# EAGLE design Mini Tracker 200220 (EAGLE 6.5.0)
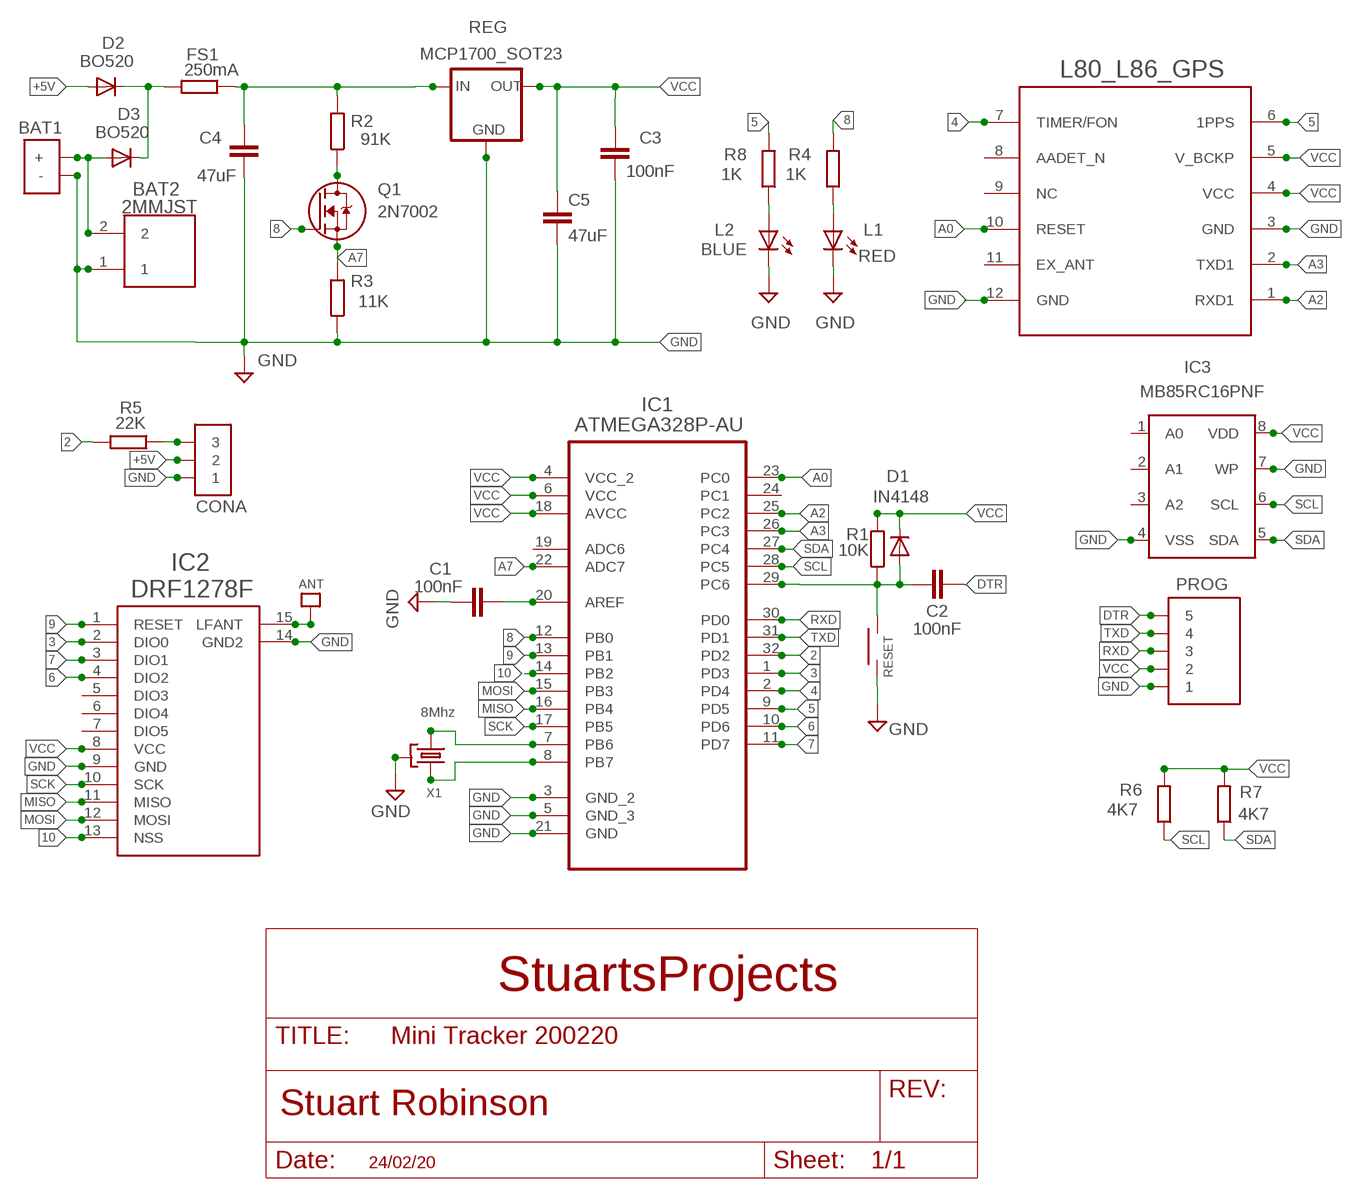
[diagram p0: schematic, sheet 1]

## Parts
ANT  SINGLEPAD  [SINGLEPAD]
BAT1  BATPADS2  [BATPADS]
BAT2  2MMJST  [2MMJST]
C1  100nF  C805_REDUCED  [C0805_REDUCED]
C2  100nF  C805_REDUCED  [C0805_REDUCED]
C3  100nF  C805_REDUCED  [C0805_REDUCED]
C4  47uF  C-EUC1206  [C1206]
C5  47uF  C-EUC1206  [C1206]
CONA  3X1  [3X1]
D1  IN4148  DIODE-SOD123  [SOD123]
D2  BO520  DIODE-SOD123  [SOD123]
D3  BO520  DIODE-SOD123  [SOD123]
FS1  250mA  R-EU_R1206  [R1206]
IC1  ATMEGA328P-AU  [QFP80P900X900X120-32N]
IC2  DRF1278F  DRF1278F_SMT  [DRF1278_SMT]
IC3  MB85RC16PNF  24L256  [SOIC08@1]
L1  RED  LEDCHIPLED_0805  [CHIPLED_0805]
L2  BLUE  LEDCHIPLED_0805  [CHIPLED_0805]
L80_L86_GPS  L80_L86  L80_GNSS_MODULE  [L80_PACKAGE]
PROG  5X1  [5X1]
Q1  2N7002  [SOT23]
R1  10K  R0805_REDUCED  [R0805_REDUCED]
R2  91K  R0805_REDUCED  [R0805_REDUCED]
R3  11K  R0805_REDUCED  [R0805_REDUCED]
R4  1K  R0805_REDUCED  [R0805_REDUCED]
R5  22K  R0805_REDUCED  [R0805_REDUCED]
R6  4K7  R0805_REDUCED  [R0805_REDUCED]
R7  4K7  R0805_REDUCED  [R0805_REDUCED]
R8  1K  R0805_REDUCED  [R0805_REDUCED]
REG  MCP1700_SOT23  [SOT23]
RESET  SMTSWITCH_4_X_3  [SMTSWITCH_4_X_3]
X1  8Mhz  SMTRESONATOR3  [SMTRESONATOR3]

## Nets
2: IC1.32(PD2) R5.2
3: IC1.1(PD3) IC2.2(DIO0)
4: IC1.2(PD4) L80_L86_GPS.7(TIMER/FON)
5: IC1.9(PD5) L80_L86_GPS.6(1PPS) R8.2
6: IC1.10(PD6) IC2.4(DIO2)
7: IC1.11(PD7) IC2.3(DIO1)
8: IC1.12(PB0) Q1.1(G) R4.2
9: IC1.13(PB1) IC2.1(RESET)
10: IC1.14(PB2) IC2.13(NSS)
+5V [POWER]: CONA.2 D2.A
A0: IC1.23(PC0) L80_L86_GPS.10(RESET)
A2: IC1.25(PC2) L80_L86_GPS.1(RXD1)
A3: IC1.26(PC3) L80_L86_GPS.2(TXD1)
A7: IC1.22(ADC7) Q1.2(S) R3.2
DTR: C2.2 PROG.5
GND [POWER]: BAT1.BAT-V(-) BAT2.1 C1.2 C3.2 C4.2 C5.2 CONA.1 IC1.3(GND_2) IC1.5(GND_3) IC1.21(GND) IC2.9(GND) IC2.14(GND2) IC3.4(VSS) IC3.7(WP) L1.C L2.C L80_L86_GPS.3(GND) L80_L86_GPS.12(GND) PROG.1 R3.1 REG.1(GND) RESET.1 X1.G(GND)
MISO: IC1.16(PB4) IC2.11(MISO)
MOSI: IC1.15(PB3) IC2.12(MOSI)
N$1: IC1.8(PB7) X1.X2
N$2: IC1.7(PB6) X1.X1
N$3: C1.1 IC1.20(AREF)
N$4: ANT.P$1 IC2.15(LFANT)
N$5 [POWER]: D2.C D3.C FS1.2
N$6: L1.A R4.1
N$8: CONA.3 R5.1
N$9: Q1.3(D) R2.1
N$11 [POWER]: C4.1 FS1.1 R2.2 REG.3(IN)
N$12 [POWER]: BAT1.BAT+(+) BAT2.2 D3.A
N$13: L2.A R8.1
RESET: C2.1 D1.A IC1.29(PC6) R1.1 RESET.2
RXD: IC1.30(PD0) PROG.3
SCK: IC1.17(PB5) IC2.10(SCK)
SCL: IC1.28(PC5) IC3.6(SCL) R6.1
SDA: IC1.27(PC4) IC3.5(SDA) R7.1
TXD: IC1.31(PD1) PROG.4
VCC [VDD]: C3.1 C5.1 D1.C IC1.4(VCC_2) IC1.6(VCC) IC1.18(AVCC) IC2.8(VCC) IC3.8(VDD) L80_L86_GPS.4(VCC) L80_L86_GPS.5(V_BCKP) PROG.2 R1.2 R6.2 R7.2 REG.2(OUT)
Unconnected: IC1.19(ADC6) IC1.24(PC1) IC2.5(DIO3) IC2.6(DIO4) IC2.7(DIO5) IC3.1(A0) IC3.2(A1) IC3.3(A2) L80_L86_GPS.8(AADET_N) L80_L86_GPS.9(NC) L80_L86_GPS.11(EX_ANT)

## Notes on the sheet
- StuartsProjects
- 24/02/20

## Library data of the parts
ANT = LMA2:SINGLEPAD
BAT1 = LMA2:BATPADS2
BAT2 = LMA2:2MMJST
C1-C3 = resistor:C805_REDUCED
C4 C5 = resistor:C-EU: CAPACITOR, European symbol
CONA = My_Pin_Headers:3X1
D1-D3 = diode:DIODE-: DIODE
FS1 = resistor:R-EU_: RESISTOR, European symbol
IC1 = atmel:ATMEGA328P-AU: 8-bit Microcontroller with In-System Programmable Flash; MPN: ATMEGA328P-AU; OC_FARNELL: 1715486; OC_NEWARK: 14R4631; PACKAGE: TQFP-32; SUPPLIER: Atmel
IC2 = LMA2:DRF1278F_SMT
IC3 = LMA2:24L256
L1 L2 = led:LED: LED
L80_L86_GPS = Quectel:L80_GNSS_MODULE: GPS module with an embedded patch antenna (15mmx15mmx4mm)
PROG = My_Pin_Headers:5X1
Q1 = LMA2:2N7002
R1-R8 = resistor:R0805_REDUCED
REG = LMA2:MCP1700_SOT23
RESET = LMA2:SMTSWITCH_4_X_3
X1 = LMA2:SMTRESONATOR3

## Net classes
0 default: width 0.152 mm
1 POWER: width 0.508 mm
2 VDD: width 0.508 mm
3 gpspower: width 0.508 mm

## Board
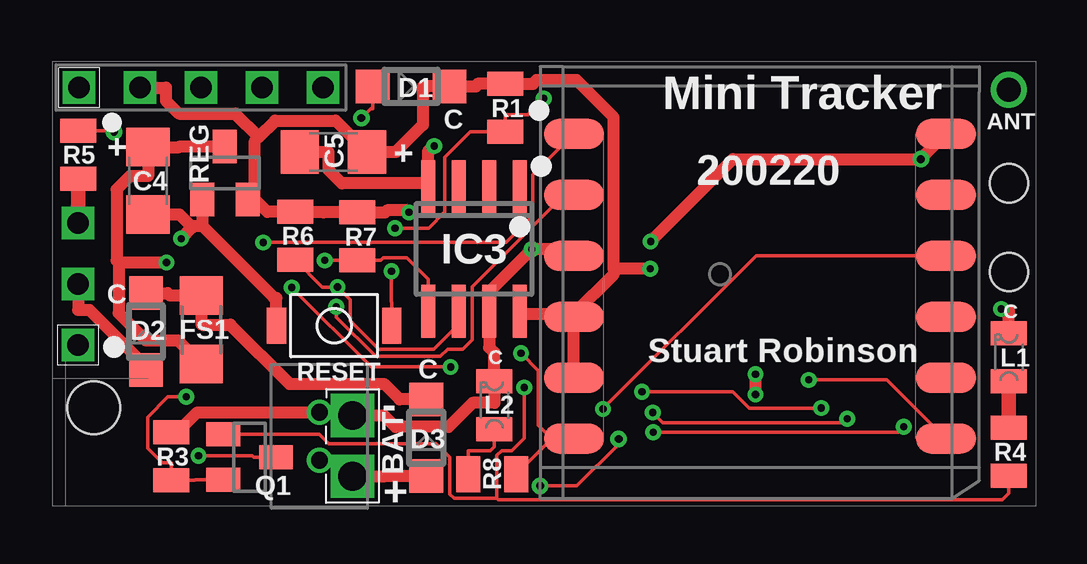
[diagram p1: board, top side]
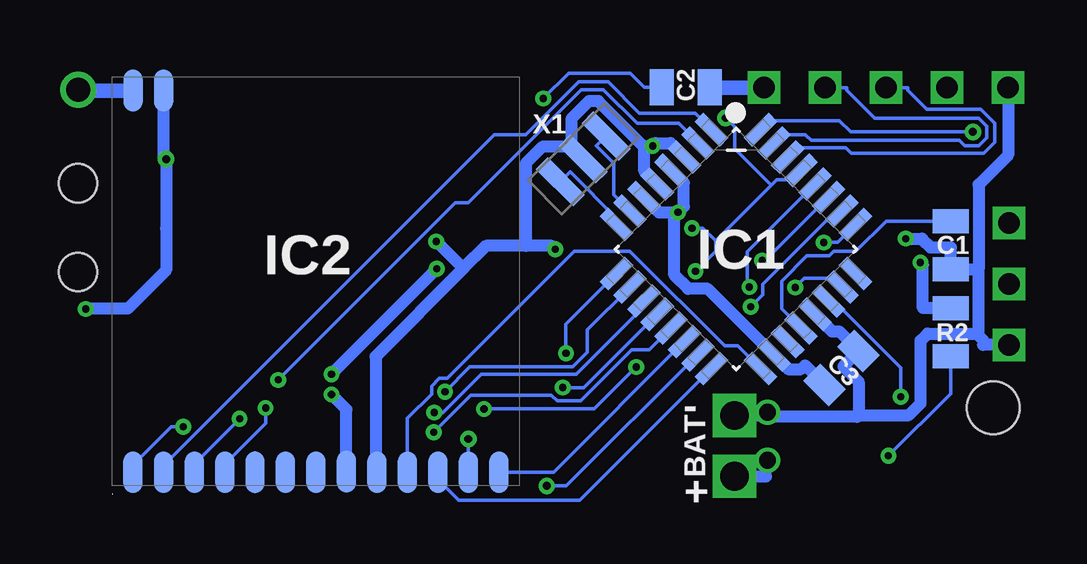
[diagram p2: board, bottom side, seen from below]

No outline drawn. Coordinates in mm, seen from the top.
Copper layers (1*16): Top 0.0356mm / dielectric 1.5011mm / Bottom 0.0356mm
Design rules "LaenPCBOrder *": minimum track width 6mil, minimum drill 13mil, track to track 6mil, track to pad 6mil, pad to pad 6mil, via to via 6mil, smd to smd 6mil, copper to edge 15mil, drill to drill 6mil, minimum pad ring 7mil, minimum via ring 7mil, stop-mask expansion 4mil, vias tented up to drill 1000mil, thermal gap 10mil
Holes 2.2 mm at 1.74,4.09
Holes 1.6 mm at 39.87,13.45 39.87,9.75
bRestrict: area 35.4,17.3 to 35.4,17.3

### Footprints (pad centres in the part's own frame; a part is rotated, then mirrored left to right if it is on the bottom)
SINGLEPAD = drill 1: P$1 0,0
BATPADS = drill 1.2 pad 1.778 square: BAT+ 0,-1.27; BAT-V 0,1.27
2MMJST = drill 0.7: 1 -1,0; 2 1,0
C0805_REDUCED = smd 1 x 1.5: 1 -1,0; 2 1,0
C1206 = smd 1.6 x 1.8: 1 -1.4,0; 2 1.4,0
3X1 = drill 0.9 square: 1 -2.54,0; 2 0,0; 3 2.54,0
SOD123 = smd 1.4 x 1.4: A 1.6,0; C -1.6,0
R1206 = smd 1.6 x 1.803: 1 -1.422,0; 2 1.422,0
QFP80P900X900X120-32N = smd 1.473 x 0.508: 1 -4.242,2.794; 2 -4.242,2.007; 3 -4.242,1.194; 4 -4.242,0.406; 5 -4.242,-0.406; 6 -4.242,-1.194; 7 -4.242,-2.007; 8 -4.242,-2.794; 17 4.242,-2.794; 18 4.242,-2.007; 19 4.242,-1.194; 20 4.242,-0.406; 21 4.242,0.406; 22 4.242,1.194; 23 4.242,2.007; 24 4.242,2.794 | smd 0.508 x 1.473: 9 -2.794,-4.242; 10 -2.007,-4.242; 11 -1.194,-4.242; 12 -0.406,-4.242; 13 0.406,-4.242; 14 1.194,-4.242; 15 2.007,-4.242; 16 2.794,-4.242; 25 2.794,4.242; 26 2.007,4.242; 27 1.194,4.242; 28 0.406,4.242; 29 -0.406,4.242; 30 -1.194,4.242; 31 -2.007,4.242; 32 -2.794,4.242
DRF1278_SMT = smd 0.8 x 1.75: 1 -1.015,-0.695; 2 -2.295,-0.695; 3 -3.575,-0.695; 4 -4.845,-0.695; 5 -6.105,-0.695; 6 -7.375,-0.695; 7 -8.645,-0.695; 8 -9.915,-0.725; 9 -11.185,-0.695; 10 -12.455,-0.695; 11 -13.725,-0.695; 12 -14.995,-0.695; 13 -16.265,-0.695; 14 -2.295,-16.595; 15 -1.025,-16.595
SOIC08@1 = smd 0.6 x 2.2: 1 -1.905,-2.6; 2 -0.635,-2.6; 3 0.635,-2.6; 4 1.905,-2.6; 5 1.905,2.6; 6 0.635,2.6; 7 -0.635,2.6; 8 -1.905,2.6
CHIPLED_0805 = smd 1.5 x 1: A 0,-1; C 0,1
L80_PACKAGE = smd 2.5 x 1.25: 1 15.75,1.8; 2 15.75,4.34; 3 15.75,6.88; 4 15.75,9.42; 5 15.75,11.96; 6 15.75,14.5; 7 0.25,14.5; 8 0.25,11.96; 9 0.25,9.42; 10 0.25,6.88; 11 0.25,4.34; 12 0.25,1.8
5X1 = drill 0.9 square: 1 -5.08,0; 2 -2.54,0; 3 0,0; 4 2.54,0; 5 5.08,0
SOT23 = smd 1 x 1.4: 1 -0.95,-1.1; 2 0.95,-1.1; 3 0,1.1
R0805_REDUCED = smd 1 x 1.5: 1 -1,0; 2 1,0
SMTSWITCH_4_X_3 = smd 0.8 x 1.5: 1 -2.4,0; 2 2.4,0
SMTRESONATOR3 = smd 0.7 x 2.2: G 0,0; X1 -1.35,0; X2 1.35,0

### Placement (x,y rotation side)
ANT  39.87,17.34 0 top
BAT1  12.52,2.5 0 top
BAT2  11.14,2.9 270 top
C1  3.5,10.87 270 bottom
C2  14.54,17.44 0 bottom
C3  8.05,5.75 45 bottom
C4  4,13.55 270 top
C5  11.72,14.75 180 top
CONA  1.08,9.25 90 top
D1  14.96,17.48 180 top
D2  3.91,7.27 270 top
D3  15.59,2.84 270 top
FS1  6.22,7.34 90 top
IC1  12.45,10.7 315 bottom
IC2  38.6,0.71 180 bottom
IC3  17.58,10.71 180 top
L1  39.87,6.19 0 top
L2  18.43,4.2 0 top
L80_L86_GPS  37.49,17.3 180 top
PROG  6.2,17.43 0 top
Q1  8.23,2.03 270 top
R1  18.88,16.58 90 top
R2  3.51,7.24 90 bottom
R3  4.96,2.06 270 top
R4  39.87,2.26 270 top
R5  1.08,14.64 90 top
R6  10.13,11.25 90 top
R7  12.72,11.23 90 top
R8  18.34,1.32 0 top
REG  7.2,13.87 0 top
RESET  11.75,7.51 0 top
X1  18.82,14.46 225 bottom

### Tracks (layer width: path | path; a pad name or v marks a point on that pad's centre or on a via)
2  (via drill 0.33 pad 0.69)
  Top 0.152: R5.2 2.52,15.64 v2.58,15.58
  Bottom 0.152: IC1.32 11.4,15.7 11.05,16.05 8.15,16.05 7.67,15.58 v2.58,15.58 | IC1.32 | IC1.32
3
  Bottom 0.152: IC2.2 36.3,1.69 22.53,15.46 21.2,15.46 19,17.67 17.79,17.67 16.48,16.36 14.16,16.36 IC1.1 | IC1.1 | IC1.1
4  (via drill 0.3 pad 0.66)
  Top 0.152: L80_L86_GPS.7 34.79,5.25 v31.53,5.25
  Bottom 0.152: v31.53,5.25 24.14,12.64 23.6,12.64 18.89,17.35 17.98,17.35 16.57,15.94 14.85,15.94 IC1.2 | IC1.2
5  (via drill 0.3 pad 0.66)
  Top 0.152: 20.82,2.8 L80_L86_GPS.6 | R8.2 20.82,2.8 | 20.82,2.8 20.26,3.36 20.26,5.64 v19.54,6.36
  Bottom 0.152: 18.35,8.75 19.54,7.56 v19.54,6.36 | 18.35,8.75 | 18.35,8.75 IC1.9
6  (via drill 0.3 pad 0.66)
  Top 0.152: v24.58,4.76 | v24.58,4.76 28.36,4.76 29.05,4.08 v32.05,4.08
  Bottom 0.152: IC2.4 33.76,1.74 32.05,3.44 v32.05,4.08 | v24.58,4.76 23.55,5.79 19.26,5.79 18.65,6.4 18.65,7.33 IC1.10 | IC1.10
7  (via drill 0.3 pad 0.66)
  Top 0.152: v33.13,3.63 32.97,3.46 25.45,3.46 v25.03,3.89
  Bottom 0.152: IC1.11 16.29,8.3 19.11,5.49 23.06,5.49 | 23.06,5.49 | 23.06,5.49 24.66,3.89 v25.03,3.89 | IC2.3 35.02,1.74 v33.13,3.63 | IC1.11 | IC1.11
8  (via drill 0.3 pad 0.66)
  Top 0.152: 18.54,0.32 18.54,2.1 18.73,2.3 19.16,2.3 19.68,2.82 v19.68,4.93 | 18.54,0.32 18.59,0.26 39.6,0.26 39.87,0.53 R4.2 | 18.54,0.32 16.75,0.32 16.58,0.49 16.58,2.02 16.01,2.59 11.53,2.59 11.14,2.98 Q1.1
  Bottom 0.152: IC1.12 18.8,4.93 v19.68,4.93 | IC1.12 | IC1.12
9  (via drill 0.3 pad 0.66)
  Top 0.152: v35.48,3.3 35.25,3.07 v25.05,3.07
  Bottom 0.152: IC1.13 16.07,6.51 16.79,6.51 18.92,4.37 19.91,4.37 20.14,4.61 23.51,4.61 v25.05,3.07 | IC2.1 37.59,1.7 35.98,3.3 v35.48,3.3 | IC1.13 | IC1.13
10
  Bottom 0.152: IC2.13 20.06,1.41 IC1.14 | IC1.14 | IC1.14
+5V
  Top 0.508: CONA.2 1.08,8.17 1.56,8.17 3.91,5.81 D2.A
A0  (via drill 0.3 pad 0.66)
  Top 0.152: L80_L86_GPS.10 29.33,10.42 v22.95,4.04 | v16.61,5.79 13.29,5.79 v9.99,9.1
  Bottom 0.152: v16.61,5.79 18.36,4.04 v22.95,4.04 | v9.99,9.1 9.61,9.48 8.39,9.48 IC1.23 | IC1.23
A2  (via drill 0.3 pad 0.66)
  Top 0.152: L80_L86_GPS.1 20.03,13.79 20.03,12.08 18.93,10.98 v8.8,10.98
  Bottom 0.152: IC1.25 8.22,10.98 v8.8,10.98 | IC1.25 | IC1.25
A3  (via drill 0.3 pad 0.66)
  Top 0.152: v11.84,8.3 11.84,7.87 13.48,6.23 16.18,6.23 16.48,6.53 17.11,6.53 17.51,6.93 17.51,9.13 21.34,12.96 L80_L86_GPS.2
  Bottom 0.152: v11.84,8.3 11.34,8.8 11.34,9.24 8.29,12.28 IC1.26 | IC1.26
A7  (via drill 0.3 pad 0.66)
  Top 0.152: v5.59,4.54 4.83,4.54 3.98,3.7 3.98,2.4 4.6,1.79 4.96,1.79 R3.2 5.94,1.06 5.96,1.08 Q1.2
  Bottom 0.152: v5.59,4.54 5.59,5.76 8.37,8.54 IC1.22 | IC1.22
DTR
  Bottom 0.61: PROG.5 C2.2
GND  (via drill 0.3 pad 0.66, 0.33 pad 0.69)
  Top 0.508: L1.C 39.87,8.1 39.65,8.1 v39.55,8.2 | v24.94,11.02 28.37,14.45 v36.2,14.45 v36.2,14.46 L80_L86_GPS.12 | 5.85,11.61 5.9,11.66 6.25,11.66 | v5.38,11.14 5.85,11.61 | 5.85,11.61 5.31,12.15 C4.2 | RESET.1 9.35,8.67 9.25,8.67 6.25,11.66 | C5.2 11.53,14.75 11.53,14 12.08,13.44 15.68,13.44 | IC3.4 15.68,13.44 | 15.68,13.44 15.68,13.54 15.68,14.82 15.75,14.82 v15.93,14.99 | BAT1.BAT-V 13.83,3.77 14.31,3.29 16.52,3.29 17.52,4.29 18.43,4.29 L2.C 18.43,6.39 18.21,6.6 IC3.7 18.21,8.92 v19.99,10.7 21.46,10.7 L80_L86_GPS.3 | REG.1 6.25,11.66 | R3.1 5.21,3.06 6.05,3.9 BAT2.1
  Bottom 0.152: IC1.3 | IC1.3 | IC1.5 | IC1.5 | IC1.21 | IC1.21 | C3.2
  Bottom 0.508: 21.21,10.84 22.87,10.84 23.81,9.89 | v19.99,10.7 20.13,10.84 21.21,10.84 | 19.32,14.96 20.52,14.96 21.21,14.27 21.21,10.84 | 19.32,14.96 X1.G | 16.27,14.99 16.32,14.99 18.18,16.86 18.59,16.86 19.32,16.13 19.32,14.96 | 23.81,9.89 v24.94,11.02 | 23.81,9.89 27.47,6.23 27.47,1.46 IC2.9 | PROG.1 1.12,14.62 2.34,13.39 2.34,9.87 | v5.38,11.14 4.71,11.14 4.35,10.78 3.5,10.78 C1.2 2.34,9.87 | 2.42,7.18 2.34,7.26 2.34,9.87 | 7.34,3.78 5.26,3.78 4.76,4.28 4.76,6.88 4.47,7.18 2.42,7.18 | 2.42,7.18 2.16,6.91 2.16,6.71 CONA.1 | IC1.5 16.27,13.95 16.27,14.99 | 16.27,14.99 v15.93,14.99 15.81,15.12 15.18,15.12 IC1.3 | BAT1.BAT-V 11.21,3.77 11.21,3.83 BAT2.1 10.95,3.71 7.41,3.71 7.34,3.78 | 7.34,3.78 7.34,5.17 7.98,5.82 C3.2 8.16,7.28 8.45,7.28 IC1.21 | IC2.14 36.3,14.55 v36.2,14.45 36.2,11.55 36.2,9.82 37.8,8.22 39.53,8.22 v39.55,8.2
MISO
  Bottom 0.152: IC2.11 24.88,1.11 24,0.24 18.96,0.24 14.4,4.8 | 14.4,4.8 | 14.4,4.8 IC1.16
MOSI  (via drill 0.33 pad 0.69)
  Top 0.152: v23.61,2.79 23.61,2.57 21.87,0.83 v20.34,0.83
  Bottom 0.152: IC2.12 v23.61,2.79 | v20.34,0.83 19.52,0.83 14.05,6.3 IC1.15 | IC1.15
N$1
  Bottom 0.152: X1.X2 | X1.X2 19.36,13.91 17.43,11.97 IC1.8 | X1.X2 | IC1.8 | IC1.8
N$2
  Bottom 0.152: X1.X1 | X1.X1 18.27,15.01 17.55,14.28 17.55,12.96 IC1.7 | IC1.7 | X1.X1
N$3
  Bottom 0.152: IC1.20 10.55,8.22 10.55,9.37 9.5,10.42 8.57,10.42 8.38,10.61 7.46,10.61 6.19,11.87 4.48,11.87 C1.1 | IC1.20 | IC1.20
N$4
  Bottom 0.152: 39.84,17.3 ANT.P$1
  Bottom 0.61: IC2.15 39.84,17.3
N$5
  Top 0.508: D3.C 14.48,4.44 13.84,5.09 9.89,5.09 7.43,7.56 6.22,7.56 FS1.2 4.91,8.76 4.8,8.87 D2.C
N$6
  Top 0.61: R4.1 L1.A
N$8
  Top 0.61: R5.1 CONA.3
N$9  (via drill 0.3 pad 0.66)
  Top 0.152: Q1.3 8.4,2.03 8.35,2.09 v6.1,2.09
  Bottom 0.152: R2.1 3.51,4.68 v6.1,2.09
N$11  (via drill 0.3 pad 0.66)
  Top 0.508: 2.77,10.14 2.77,8.04 3.91,6.89 5.24,6.89 FS1.1 | 2.77,10.14 2.69,10.22 2.69,13.19 3.25,13.74 4,13.74 C4.1 5.31,14.95 5.33,14.97 REG.3 | 2.77,10.14 v4.77,10.14
  Bottom 0.508: v4.77,10.14 4.67,10.04 4.67,8.24 R2.2
N$12
  Top 0.508: BAT1.BAT+ 13.83,1.23 13.84,1.24 D3.A
  Bottom 0.508: BAT1.BAT+ 11.21,1.23 11.21,1.83 BAT2.2
N$13
  Top 0.152: L2.A 18.43,2.47 18.26,2.3 17.34,2.3 R8.1
RESET  (via drill 0.3 pad 0.66, 0.33 pad 0.69)
  Top 0.152: RESET.2 14.15,8.49 14.14,8.5 v14.14,9.78 | v20.49,16.98 19.82,16.31 18.88,16.31 R1.1 17.42,15.58 16.36,14.53 16.36,12.25 15.69,11.57 v14.28,11.57 | D1.A 13.36,16.55 13.27,16.55 v12.89,16.16
  Bottom 0.152: 13.3,11.05 10.99,13.36 | 10.99,13.36 10.76,13.59 10.13,13.59 IC1.29 | v14.28,11.57 13.83,11.57 13.3,11.05 | v14.14,9.78 13.3,10.62 13.3,11.05 | v20.49,16.98 19.43,18.03 16.86,18.03 16.27,17.44 C2.1 | v12.89,16.16 12.52,15.79 12.51,15.79 12.51,14.99 12.51,14.88 10.99,13.36 | IC1.29 | IC1.29
RXD
  Bottom 0.152: PROG.3 5.3,17.43 5.3,17.32 4.51,16.53 2.26,16.53 1.67,15.94 1.67,15.16 2.14,14.7 7.65,14.7 7.88,14.93 9.91,14.93 IC1.30 | IC1.30
SCK
  Bottom 0.152: IC2.10 26.14,3.65 25.14,4.66 25.14,4.99 24.81,5.32 24.48,5.32 19.18,10.61 16.88,10.61 16.78,10.51 16.77,10.51 12.93,6.67 12.37,6.67 IC1.17
SCL  (via drill 0.3 pad 0.66)
  Top 0.152: IC3.6 16.95,7.58 15.9,6.53 13.61,6.53 12.42,7.71 12.42,8.59 v11.89,9.12 11.26,9.12 R6.1
  Bottom 0.152: v11.89,9.12 11.98,9.21 11.98,10.59 IC1.28 | IC1.28 | IC1.28
SDA  (via drill 0.3 pad 0.66)
  Top 0.152: IC3.5 15.68,9.44 14.78,10.33 13.8,10.33 13.7,10.23 R7.1 v11.36,10.23
  Bottom 0.152: v11.36,10.23 11.23,10.23 IC1.27 | IC1.27
TXD
  Bottom 0.152: PROG.4 7.84,17.43 7.84,17.32 6.67,16.15 2.34,16.15 2.01,15.82 2.01,15.34 2.35,15 2.92,15 3.15,15.23 9.31,15.23 9.56,15.47 10.51,15.47 IC1.31 | IC1.31
VCC  (via drill 0.3 pad 0.66)
  Top 0.508: v29.31,4.64 v29.31,5.49 | 21.74,7.98 19.62,7.98 IC3.8 | 23.4,9.88 23.4,9.64 21.74,7.98 | 21.74,7.98 L80_L86_GPS.4 L80_L86_GPS.5 | 23.4,9.88 23.4,16.19 21.85,17.74 20.19,17.74 20.04,17.58 R1.2 17.72,17.58 17.72,17.54 17.67,17.48 D1.C 15.45,17.48 15.45,15.88 14.33,14.75 C5.1 11.81,16.06 9.3,16.06 8.61,15.37 | v24.92,9.88 23.4,9.88 | 8.45,12.77 8.45,15.21 8.61,15.37 | 8.61,15.37 7.63,16.35 5.28,16.35 4.74,16.89 4.74,17.43 PROG.2 | 8.45,12.77 8.97,12.25 R6.2 11.29,12.25 11.31,12.23 R7.2 13.88,12.23 13.96,12.31 14.79,12.31 v14.87,12.23 | REG.2 8.45,12.77
  Bottom 0.152: IC1.4 | IC1.4 | IC1.6 | IC1.6 | IC1.18 | IC1.18 | C3.1
  Bottom 0.508: v14.87,12.23 15.02,12.09 15.02,9.62 14.45,9.04 13.63,9.04 IC1.18 10.29,5.7 9.74,5.7 9.57,5.86 C3.1 | v24.92,9.88 v29.31,5.49 | IC2.8 28.68,4.02 v29.31,4.64 | IC1.6 15.67,12.23 v14.87,12.23 | v14.87,12.23 14.63,12.47 14.63,13.45 IC1.4

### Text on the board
tNames: D1 | Mini Tracker | C | R1 | REG | C5 | ANT | + | + | 200220 | R5 | C4 | R6 | R7 | IC3 | C | C | D2 | FS1 | C | Stuart Robinson | L1 | C | RESET | L2 | - | R3 | D3 | R4 | BAT | R8 | Q1 | +
bNames: C2 | X1 | C1 | IC1 | IC2 | R2 | C3 | BAT | - | +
